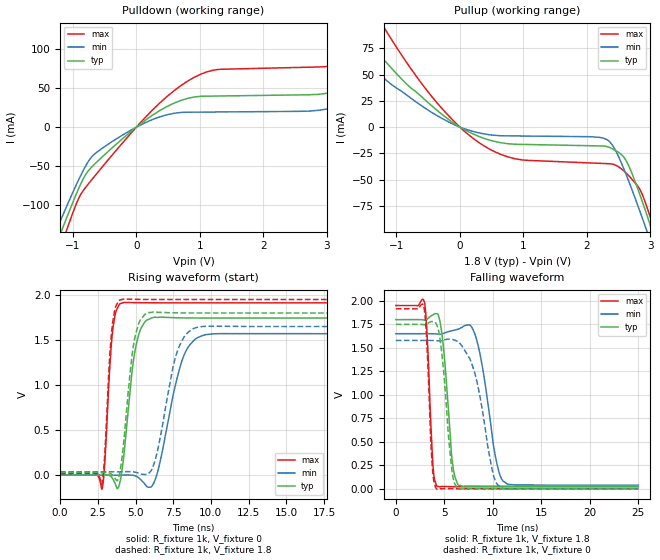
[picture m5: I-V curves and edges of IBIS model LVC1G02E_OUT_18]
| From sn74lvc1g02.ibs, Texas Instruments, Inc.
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[Model]   LVC1G02E_OUT_18
Model_type  Output
Vref =   0
Rref =   1000
Cref =   30p
Vmeas =   0.9
| variable   typ   min   max
C_comp   8.61pF   1.01pF   17.70pF
| C_pullup   4.97pF   1.01pF   7.65pF
| C_pulldown   12.24pF   6.60pF   17.70pF
[Temperature Range]   40   100   -40
| Ambient temperature   25   85   -40
[Voltage range]   1.8   1.65   1.95
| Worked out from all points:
|   slope of the pulldown table from 0 to 0.27 V, typ, clamps not added: 16.6 ohm
|   slope of the pullup table from 0 to 0.27 V, typ, clamps not added: 33.1 ohm
|   rising waveform, R_fixture 1k, V_fixture 0: 20-80 % time 679ps typ, 1.22ns min, 395ps max; typ from 0 V to 1.74 V
|   falling waveform, R_fixture 1k, V_fixture 1.8: 20-80 % time 762ps typ, 1.37ns min, 483ps max; typ from 1.8 V to 0.027 V
|   rising waveform, R_fixture 1k, V_fixture 1.8: 20-80 % time 644ps typ, 1.11ns min, 383ps max; typ from 0.027 V to 1.8 V
|   falling waveform, R_fixture 1k, V_fixture 0: 20-80 % time 840ps typ, 1.67ns min, 465ps max; typ from 1.75 V to 0 V
[Pulldown]
| LVC1G02E_OUT_18
|   Voltage   I(typ)   I(min)   I(max)
-5.5V     -1.048A    -958.1mA   -1.163A
-1.25V    -148.5mA   -130.6mA   -168.3mA
-1.095V   -116mA     -101.3mA   -131.7mA
-640mV    -46.19mA   -33.33mA   -61.35mA
810mV     37.05mA    19.18mA    59.31mA
3.12V     45.59mA    25.26mA    79.75mA
3.755V    64.52mA    35.93mA    102.7mA
4.215V    79.1mA     21.54mA    129.8mA
4.445V    47.14mA    21.67mA    144.7mA
4.725V    44.49mA    21.83mA    131.7mA
5.01V     44.71mA    22mA       83.05mA
11V       50.72mA    25.33mA    92.94mA
[Pullup]
| LVC1G02E_OUT_18
|   Voltage   I(typ)   I(min)   I(max)
-5.5V     480.5mA    377.4mA    671.8mA
-2.005V   126.2mA    94.48mA    183.1mA
-1.63V    95.94mA    70.94mA    140.4mA
-1.275V   69.59mA    50.71mA    102.9mA
-275mV    11.83mA    8.035mA    17.18mA
435mV     -11.75mA   -6.982mA   -19.84mA
985mV     -16.42mA   -8.45mA    -31.22mA
2.32V     -18.58mA   -12.07mA   -34.74mA
2.615V    -31.69mA   -44.77mA   -43.53mA
2.94V     -82.86mA   -98.13mA   -75.18mA
3.075V    -107.5mA   -121.6mA   -100.6mA
11V       -1.752A    -1.655A    -1.883A
[Ramp]
| LVC1G02E_OUT_18
| variable   typ   min   max
dV/dt_r   1.14/7.63E-10   1.02/1.32E-09   1.24/4.35E-10
dV/dt_f   1.10/8.23E-10   1.02/1.52E-09   1.20/5.16E-10
R_load = 1k
[Rising Waveform]
| LVC1G02E_OUT_18
R_fixture =   1k
C_fixture =   0
L_fixture =   0
V_fixture =   0
V_fixture_min = 0
V_fixture_max = 0
|   Time   V(typ)   V(min)   V(max)
0s        112.7pV    7.663nV    3.037nV
2.785ns   22.59uV    -20.77uV   -147.8mV
3.45ns    -30.79mV   -94.78uV   1.552V
4.01ns    -43.69mV   478.3uV    1.907V
4.94ns    1.356V     -3.97mV    1.915V
5.78ns    1.725V     -130mV     1.914V
6.46ns    1.751V     33.18mV    1.913V
8.07ns    1.746V     1.267V     1.913V
9.105ns   1.744V     1.526V     1.913V
24.99ns   1.744V     1.569V     1.913V
[Falling Waveform]
| LVC1G02E_OUT_18
R_fixture =   1k
C_fixture =   0
L_fixture =   0
V_fixture =   1.8
V_fixture_min = 1.65
V_fixture_max = 1.95
|   Time   V(typ)   V(min)   V(max)
0s        1.8V       1.65V      1.95V
2.975ns   1.795V     1.65V      1.972V
3.8ns     1.849V     1.649V     284.7mV
4.25ns    1.862V     1.647V     24.33mV
4.895ns   1.519V     1.653V     23.46mV
5.84ns    275.7mV    1.683V     21.51mV
6.47ns    35.46mV    1.7V       20.92mV
8.285ns   28.3mV     1.603V     21.06mV
11.09ns   27.05mV    77.76mV    21.09mV
24.99ns   26.98mV    37.17mV    21.09mV
[Rising Waveform]
| LVC1G02E_OUT_18
R_fixture =   1k
C_fixture =   0
L_fixture =   0
V_fixture =   1.8
V_fixture_min = 1.65
V_fixture_max = 1.95
|   Time   V(typ)   V(min)   V(max)
0s        26.95mV    37.1mV     21.07mV
2.77ns    26.91mV    37.09mV    -98.12mV
3.425ns   7.299mV    37.03mV    1.608V
3.975ns   48.61mV    37.4mV     1.946V
4.885ns   1.464V     35.61mV    1.952V
5.75ns    1.8V       8.466mV    1.951V
6.405ns   1.809V     233.9mV    1.95V
7.725ns   1.802V     1.351V     1.95V
8.83ns    1.8V       1.627V     1.95V
24.99ns   1.8V       1.65V      1.95V
[Falling Waveform]
| LVC1G02E_OUT_18
R_fixture =   1k
C_fixture =   0
L_fixture =   0
V_fixture =   0
V_fixture_min = 0
V_fixture_max = 0
|   Time   V(typ)   V(min)   V(max)
0s        1.749V     1.578V     1.916V
2.885ns   1.746V     1.578V     1.933V
3.175ns   1.75V      1.578V     1.595V
3.755ns   1.78V      1.578V     246mV
4.2ns     1.747V     1.576V     -2.679mV
5.795ns   182.8mV    1.589V     233uV
6.395ns   3.31mV     1.566V     -168.9uV
8.105ns   609.9uV    1.242V     -4.42uV
10.8ns    52.31uV    14.08mV    18.29uV
24.99ns   22.49uV    47.99uV    13.93uV
